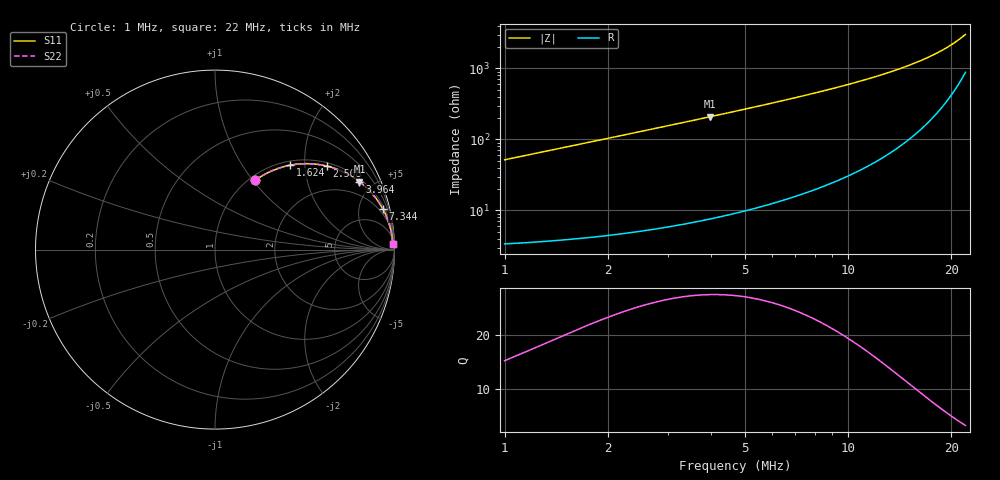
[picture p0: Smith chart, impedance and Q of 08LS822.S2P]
! Coilcraft 0805LS-822 Chip Inductor
! 18 September 2002
# MHZ S MA R 50
!Freq  MagS11  AngS11  MagS21  AngS21  MagS12  AngS12  MagS22  AngS22
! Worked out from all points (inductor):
!   405 points, 1 MHz to 22 MHz, reference 50 ohm
!   read as one part in series: L = 8.23 uH near 1.104 MHz
!   highest Q = 27.6 at 3.964 MHz (marker M1), where L = 8.37 uH
!   S11 on the Smith chart (normalised r, x): 1 MHz: 1.07, +1.03; 1.624 MHz: 1.08, +1.68; 2.508 MHz: 1.10, +2.61; 3.964 MHz: 1.15, +4.17; 7.344 MHz: 1.34, +8.14; 22 MHz: 19, +58
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1  0.4475 59.7  0.8656 -26.5  0.8656 -26.5  0.4475 59.7
1.104  0.4832 57.7  0.8467 -28.8  0.8467 -28.8  0.4832 57.7
1.364  0.5626 52.8  0.7976 -34.2  0.7976 -34.2  0.5626 52.8
1.624  0.6289 48.4  0.7482 -38.9  0.7482 -38.9  0.6289 48.4
2.04  0.7117 42.2  0.6729 -45.3  0.6729 -45.3  0.7117 42.2
2.508  0.7788 36.7  0.5974 -51.1  0.5974 -51.1  0.7788 36.7
2.82  0.8124 33.5  0.553 -54.3  0.553 -54.3  0.8124 33.5
3.184  0.8434 30.4  0.507 -57.4  0.507 -57.4  0.8434 30.4
3.548  0.8676 27.8  0.4666 -60.1  0.4666 -60.1  0.8676 27.8
3.964  0.8893 25.2  0.4262 -62.7  0.4262 -62.7  0.8893 25.2
4.536  0.9116 22.3  0.3793 -65.6  0.3793 -65.6  0.9116 22.3
5.108  0.9278 19.9  0.3403 -68.0  0.3403 -68.0  0.9278 19.9
5.784  0.9419 17.6  0.302 -70.3  0.302 -70.3  0.9419 17.6
7.344  0.962 13.6  0.2361 -74.0  0.2361 -74.0  0.962 13.6
8.02  0.9675 12.4  0.2142 -75.2  0.2142 -75.2  0.9675 12.4
9.632  0.9765 9.9  0.1726 -77.2  0.1726 -77.2  0.9765 9.9
11.504  0.9825 7.8  0.1368 -78.8  0.1368 -78.8  0.9825 7.8
15.04  0.988 5.1  0.0895 -79.7  0.0895 -79.7  0.988 5.1
16.964  0.9893 4.0  0.07041 -79.2  0.07041 -79.2  0.9893 4.0
18.524  0.9898 3.2  0.05714 -78.1  0.05714 -78.1  0.9898 3.2
20.24  0.99 2.5  0.04433 -75.7  0.04433 -75.7  0.99 2.5
22  0.9899 1.8  0.03282 -71.2  0.03282 -71.2  0.9899 1.8
